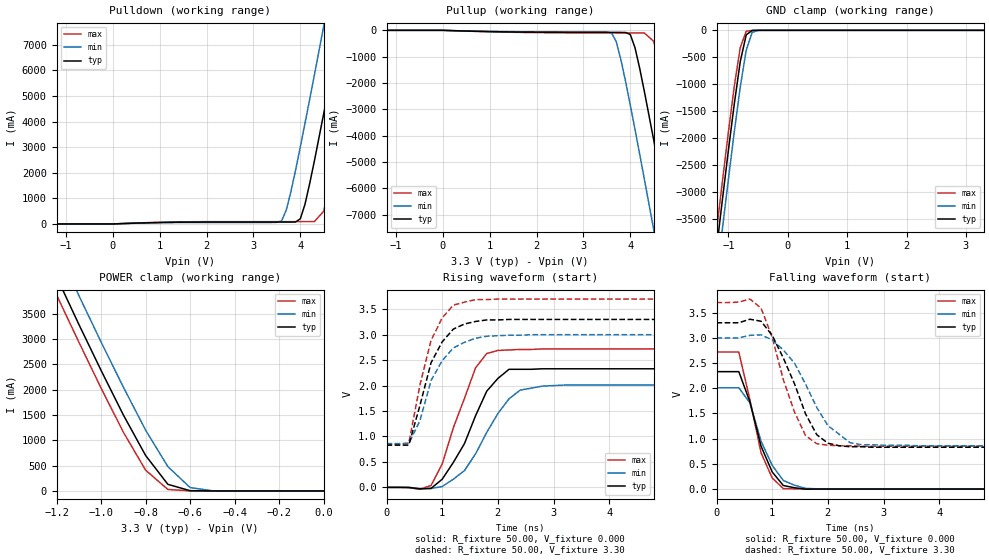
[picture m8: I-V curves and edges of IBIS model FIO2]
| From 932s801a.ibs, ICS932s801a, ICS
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|   Model FIO2
[Model]   FIO2
Model_type   I/O
Polarity   Non-Inverting
Enable   Active-High
Vinl =   0.80V
Vinh =   2.00V
C_comp   5.50pF   5.00pF   6.00pF
[Temperature Range]   27.00   70.00   0.000
[Voltage Range]   3.30V   3.00V   3.70V
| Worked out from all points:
|   slope of the pulldown table from 0 to 0.495 V, typ, clamps not added: 15.1 ohm
|   slope of the pullup table from 0 to 0.495 V, typ, clamps not added: 18.6 ohm
|   GND clamp passes 1 mA (typ) near -0.53 V on its own axis
|   POWER clamp passes 1 mA (typ) near -0.52 V on its own axis
|   rising waveform, R_fixture 50.00, V_fixture 0.000: 20-80 % time 604ps typ, 665ps min, 518ps max; typ from 0 V to 2.33 V
|   rising waveform, R_fixture 50.00, V_fixture 3.30: 20-80 % time 447ps typ, 475ps min, 413ps max; typ from 0.83 V to 3.3 V
|   falling waveform, R_fixture 50.00, V_fixture 0.000: 20-80 % time 395ps typ, 418ps min, 356ps max; typ from 2.33 V to 0 V
|   falling waveform, R_fixture 50.00, V_fixture 3.30: 20-80 % time 573ps typ, 640ps min, 488ps max; typ from 3.3 V to 0.83 V
[Pulldown]
| voltage   I(typ)   I(min)   I(max)
-3.3V     0A         0A         0A
3.6V      73.9mA     120mA      91.09mA
3.7V      73.96mA    540mA      91.15mA
4V        200mA      3.01A      91.37mA
4.1V      770mA      3.93A      91.47mA
4.3V      2.46A      5.82A      92.18mA
4.5V      4.32A      7.74A      500mA
4.7V      6.23A      9.68A      2.13A
4.9V      8.16A      11.63A     3.98A
5.1V      10.11A     13.59A     5.89A
5.3V      12.07A     15.56A     7.83A
6.6V      24.93A     28.42A     20.65A
[Pullup]
| voltage   I(typ)   I(min)   I(max)
-3.3V     0A         0A         0A
3.6V      -78.73mA   -100mA     -99.04mA
3.7V      -79.02mA   -430mA     -99.39mA
4V        -160mA     -2.84A     -100mA
4.1V      -660mA     -3.76A     -100mA
4.3V      -2.32A     -5.65A     -100mA
4.5V      -4.17A     -7.57A     -420mA
4.7V      -6.08A     -9.51A     -2A
4.9V      -8.02A     -11.46A    -3.85A
5.1V      -9.97A     -13.42A    -5.76A
5.3V      -11.93A    -15.39A    -7.7A
6.6V      -24.8A     -28.27A    -20.53A
[GND_clamp]
| voltage   I(typ)   I(min)   I(max)
-3.3V     -24.6A     -25.11A    -24.29A
-1.2V     -4.07A     -4.62A     -3.73A
-1.1V     -3.14A     -3.68A     -2.8A
-1V       -2.23A     -2.77A     -1.89A
-900mV    -1.36A     -1.88A     -1.03A
-800mV    -580mA     -1.05A     -320mA
-700mV    -83.06mA   -370mA     -17.16mA
-600mV    -2.73mA    -38.34mA   -520uA
-500mV    -100uA     -1.57mA    -32.89uA
3.3V      6.71pA     3.28uA     590fA
[POWER_clamp]
| voltage   I(typ)   I(min)   I(max)
-3.3V     24.77A     25.3A      24.44A
-1.2V     4.23A      4.8A       3.87A
-1.1V     3.29A      3.86A      2.94A
-1V       2.38A      2.94A      2.03A
-900mV    1.5A       2.05A      1.16A
-800mV    700mA      1.2A       410mA
-700mV    130mA      480mA      28.75mA
-600mV    4.44mA     65.65mA    470uA
-500mV    96.04uA    2.77mA     7.08uA
0V        6.71pA     320pA      720fA
[Ramp]
| variable   typ   min   max
dV/dt_r   1.40/0.54n   1.21/0.65n   1.63/0.43n
dV/dt_f   1.48/0.48n   1.28/0.60n   1.71/0.41n
R_load = 50.00
[Rising Waveform]
R_fixture = 50.00
V_fixture = 0.000
V_fixture_min = 0.000
V_fixture_max = 0.000
| time   V(typ)   V(min)   V(max)
0s        0V         0V         0V
800ps     -19.9mV    -21.34mV   36.82mV
1ns       160mV      16.4mV     460mV
1.2ns     490mV      160mV      1.17V
1.6ns     1.41V      660mV      2.35V
1.8ns     1.89V      1.08V      2.63V
2ns       2.14V      1.45V      2.69V
2.4ns     2.32V      1.91V      2.71V
2.8ns     2.33V      1.99V      2.72V
10ns      2.33V      2.01V      2.72V
[Rising Waveform]
R_fixture = 50.00
V_fixture = 3.30
V_fixture_min = 3.00
V_fixture_max = 3.70
| time   V(typ)   V(min)   V(max)
0s        830mV      860mV      850mV
400ps     830mV      860mV      870mV
600ps     1.61V      1.31V      2.01V
800ps     2.45V      2.1V       2.89V
1ns       2.86V      2.49V      3.33V
1.2ns     3.11V      2.74V      3.58V
1.4ns     3.21V      2.85V      3.64V
1.8ns     3.29V      2.97V      3.69V
2.6ns     3.3V       3V         3.7V
10ns      3.3V       3V         3.7V
[Falling Waveform]
R_fixture = 50.00
V_fixture = 0.000
V_fixture_min = 0.000
V_fixture_max = 0.000
| time   V(typ)   V(min)   V(max)
0s        2.33V      2.01V      2.72V
400ps     2.33V      2.01V      2.72V
600ps     1.73V      1.71V      1.77V
800ps     850mV      950mV      720mV
1ns       340mV      470mV      220mV
1.2ns     70.3mV     170mV      9.5mV
1.4ns     26.51mV    76.55mV    5.48mV
1.6ns     -1.75mV    13.26mV    2.85mV
1.8ns     1.32mV     5.8mV      1.1mV
10ns      4.04uV     4.58uV     -6.19uV
[Falling Waveform]
R_fixture = 50.00
V_fixture = 3.30
V_fixture_min = 3.00
V_fixture_max = 3.70
| time   V(typ)   V(min)   V(max)
0s        3.3V       3V         3.7V
600ps     3.37V      3.05V      3.77V
800ps     3.33V      3.06V      3.59V
1ns       3.05V      2.96V      3.01V
1.4ns     2.09V      2.5V       1.53V
1.6ns     1.49V      2.08V      1.06V
1.8ns     1.08V      1.62V      900mV
2ns       910mV      1.26V      870mV
2.6ns     840mV      880mV      850mV
10ns      830mV      860mV      850mV
